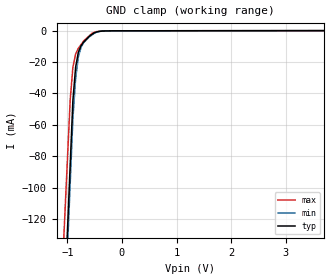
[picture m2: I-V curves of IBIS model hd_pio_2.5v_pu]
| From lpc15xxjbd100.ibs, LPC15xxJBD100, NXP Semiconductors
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[Model] hd_pio_2.5v_pu
Model_type Input
Vinl = 990.000mV
Vinh = 2.31000V
C_comp 598.000fF 598.000fF 598.000fF
| variable typ   min   max
[Voltage Range] 2.50000V 2.25000V 2.75000V
[POWER Clamp Reference] 2.50000V 2.25000V 2.75000V
[GND Clamp Reference] 0.00000V 0.00000V 0.00000V
[Temperature Range]   25   85   -40
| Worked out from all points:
|   GND clamp passes 1 mA (typ) near -0.47 V on its own axis
[GND Clamp]
-2.5V     -1.378A    -1.395A    -1.206A
-950mV    -86.18mA   -97.97mA   -44.49mA
-900mV    -44.52mA   -56.15mA   -23.31mA
-850mV    -23.34mA   -30.63mA   -14.9mA
-800mV    -13.73mA   -16.78mA   -11.26mA
-750mV    -9.608mA   -10.58mA   -8.859mA
-700mV    -7.137mA   -7.544mA   -6.459mA
-550mV    -2.299mA   -2.73mA    -1.744mA
-500mV    -1.317mA   -1.508mA   -934.4uA
-400mV    -395.5uA   -439.3uA   -349.8uA
-175mV    -86.62uA   -96.6uA    -87.06uA
5V        47.85uA    51.29uA    29.57uA
[POWER Clamp]
-2.5V     0A         0A         0A
5V        0A         0A         0A
